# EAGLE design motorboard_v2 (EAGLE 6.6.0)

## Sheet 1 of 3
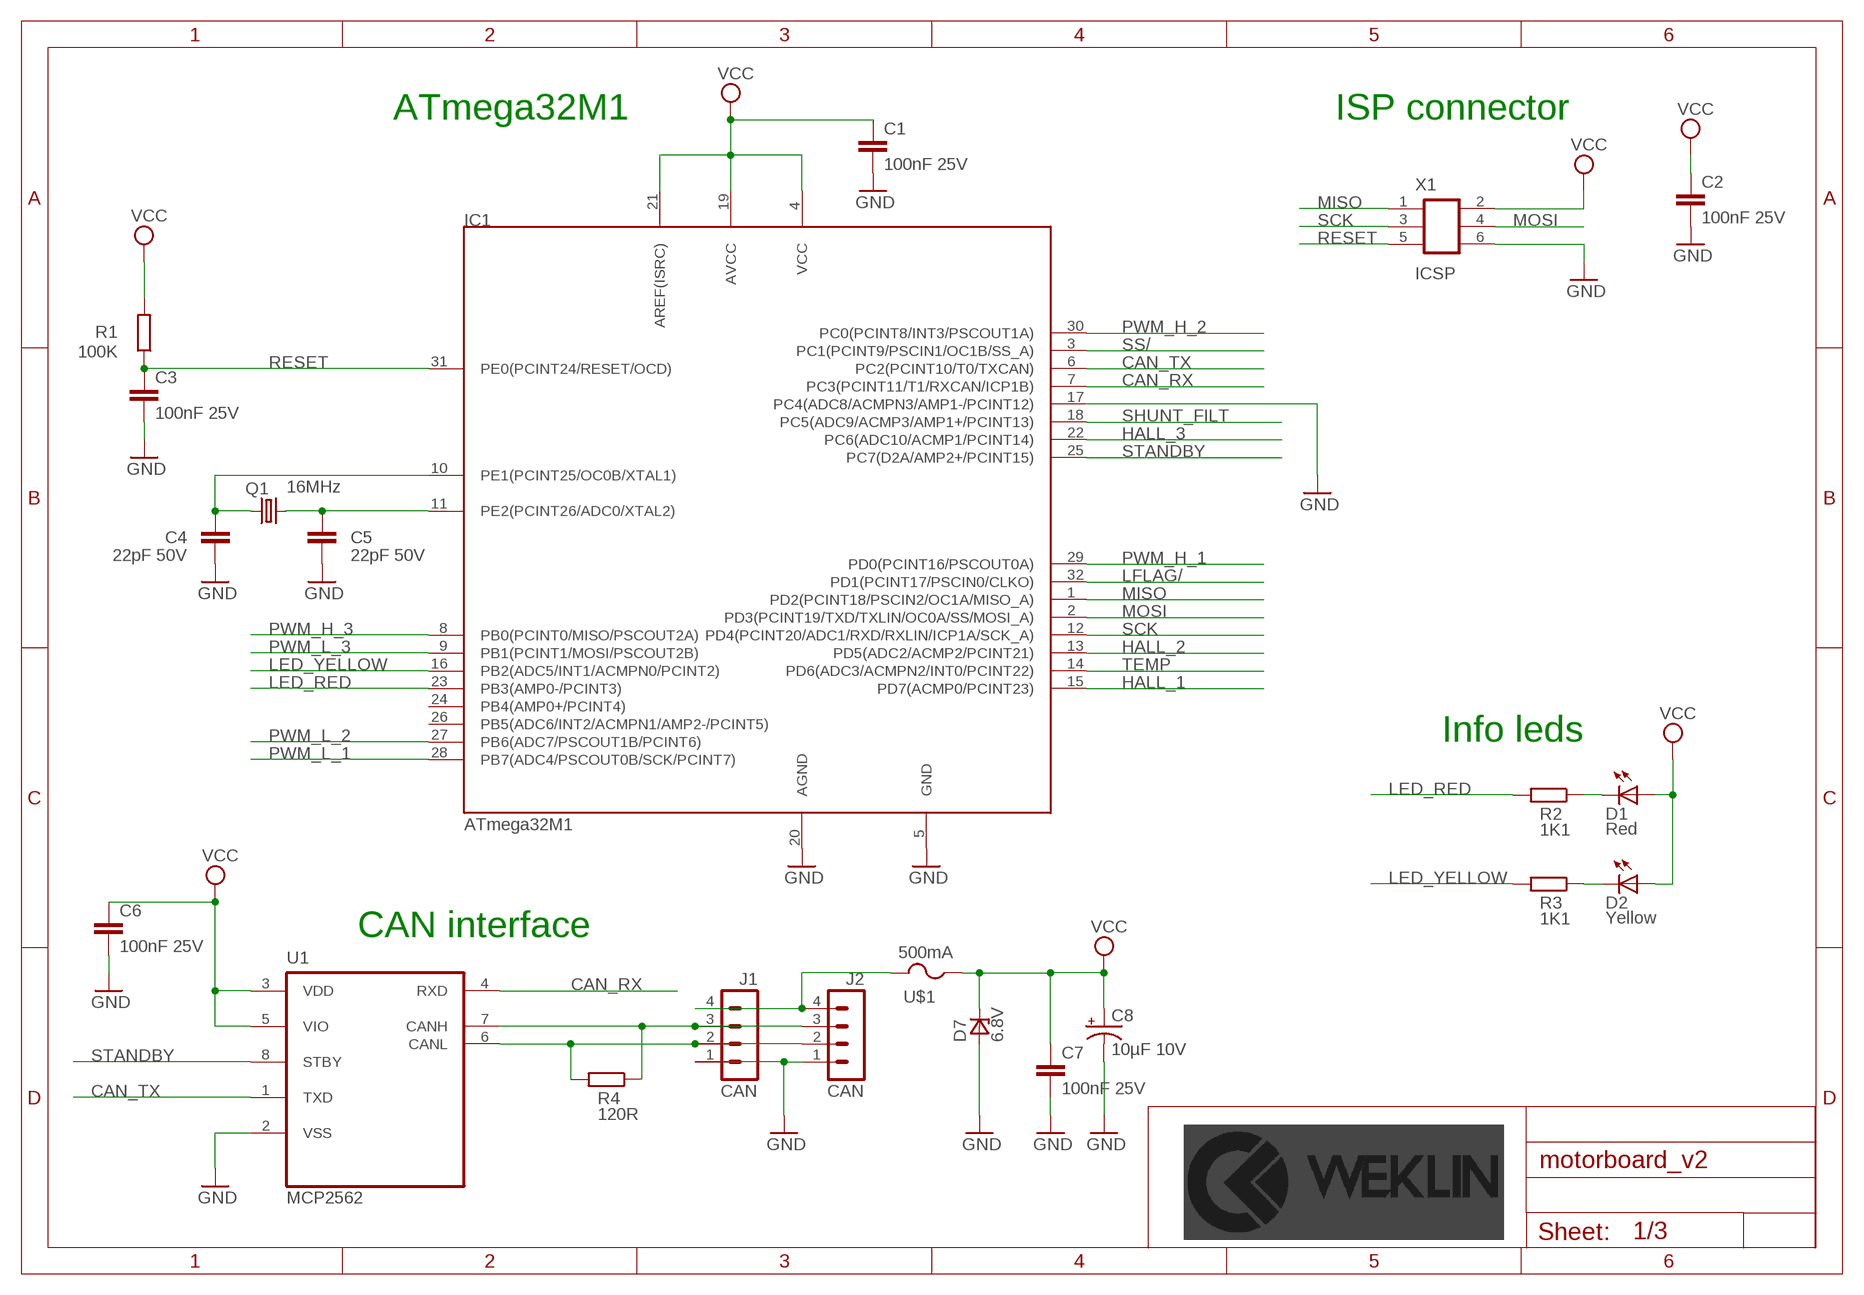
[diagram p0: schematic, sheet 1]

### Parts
C1  100nF 25V  CAPACITOR_NON_POL-100NF-25V(+-10%)(2012)  [C2012]
C2  100nF 25V  CAPACITOR_NON_POL-100NF-25V(+-10%)(2012)  [C2012]
C3  100nF 25V  CAPACITOR_NON_POL-100NF-25V(+-10%)(2012)  [C2012]
C4  22pF 50V  CAPACITOR_NON_POL-22PF-50V(+-5%)(2012)  [C2012]
C5  22pF 50V  CAPACITOR_NON_POL-22PF-50V(+-5%)(2012)  [C2012]
C6  100nF 25V  CAPACITOR_NON_POL-100NF-25V(+-10%)(2012)  [C2012]
C7  100nF 25V  CAPACITOR_NON_POL-100NF-25V(+-10%)(2012)  [C2012]
C8  10µF 10V  CAPACITOR_POL-10µF-10V(+-10%)(3216)  [EIA3216]
D1  Red  LEDVLDS1235G  [VLD]
D2  Yellow  LED-VLDY1235G  [VLD]
D7  6.8V  ZENER_UNIDIR6.8  [DO-214AA]
IC1  ATmega32M1  ATMEGA32M1-TQFP32  [TQFP32]
J1  CAN  MICROLOCK-4CMS_HORIZONTAL  [504195-0470]
J2  CAN  MICROLOCK-4CMS_HORIZONTAL  [504195-0470]
Q1  16MHz  CRYSTAL-16MHZ_SMD(3225)  [SMD_KX7]
R1  100K  RESISTOR-100K(+-1%)(2012)  [R2012]
R2  1K1  RESISTOR-1K1(+-1%)(2012)  [R2012]
R3  1K1  RESISTOR-1K1(+-1%)(2012)  [R2012]
R4  120R  RESISTOR-120R(+-1%)(2012)  [R2012]
U1  MCP2562  MCP2562-E/SN-SOIC8  [SOIC8]
U$1  500mA  FUSE0451.500MRL  [EIARS-481-2]
X1  ICSP  CON_2X3-SMD_1.27MM_FEMALE  [2X3_1.27_FEMALE_SMD]

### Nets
CAN_RX: IC1.7(PC3(PCINT11/T1/RXCAN/ICP1B)) U1.4(RXD)
CAN_TX: IC1.6(PC2(PCINT10/T0/TXCAN)) U1.1(TXD)
GND: C1.2 C2.2 C3.2 C4.2 C5.2 C6.2 C7.2 C8.C(-) D7.A IC1.5(GND) IC1.17(PC4(ADC8/ACMPN3/AMP1-/PCINT12)) IC1.20(AGND) J1.1 J2.1 U1.2(VSS) X1.6 ; also sheet 2,3
HALL_1: IC1.15(PD7(ACMP0/PCINT23)) ; also sheet 2
HALL_2: IC1.13(PD5(ADC2/ACMP2/PCINT21)) ; also sheet 2
HALL_3: IC1.22(PC6(ADC10/ACMP1/PCINT14)) ; also sheet 2
LED_RED: IC1.23(PB3(AMP0-/PCINT3)) R2.2
LED_YELLOW: IC1.16(PB2(ADC5/INT1/ACMPN0/PCINT2)) R3.2
LFLAG/: IC1.32(PD1(PCINT17/PSCIN0/CLKO)) ; also sheet 2
MISO: IC1.1(PD2(PCINT18/PSCIN2/OC1A/MISO_A)) X1.1 ; also sheet 2
MOSI: IC1.2(PD3(PCINT19/TXD/TXLIN/OC0A/SS/MOSI_A)) X1.4 ; also sheet 2
N$2: D1.C R2.1
N$3: D2.C R3.1
N$4: J1.4 J2.4 U$1.2
N$5: J1.2 J2.2 R4.2 U1.6(CANL)
N$6: J1.3 J2.3 R4.1 U1.7(CANH)
N$7: C5.1 IC1.11(PE2(PCINT26/ADC0/XTAL2)) Q1.3
N$9: C4.1 IC1.10(PE1(PCINT25/OC0B/XTAL1)) Q1.1
PWM_H_1: IC1.29(PD0(PCINT16/PSCOUT0A)) ; also sheet 3
PWM_H_2: IC1.30(PC0(PCINT8/INT3/PSCOUT1A)) ; also sheet 3
PWM_H_3: IC1.8(PB0(PCINT0/MISO/PSCOUT2A)) ; also sheet 3
PWM_L_1: IC1.28(PB7(ADC4/PSCOUT0B/SCK/PCINT7)) ; also sheet 3
PWM_L_2: IC1.27(PB6(ADC7/PSCOUT1B/PCINT6)) ; also sheet 3
PWM_L_3: IC1.9(PB1(PCINT1/MOSI/PSCOUT2B)) ; also sheet 3
RESET: C3.1 IC1.31(PE0(PCINT24/RESET/OCD)) R1.1 X1.5
SCK: IC1.12(PD4(PCINT20/ADC1/RXD/RXLIN/ICP1A/SCK_A)) X1.3 ; also sheet 2
SHUNT_FILT: IC1.18(PC5(ADC9/ACMP3/AMP1+/PCINT13)) ; also sheet 2
SS/: IC1.3(PC1(PCINT9/PSCIN1/OC1B/SS_A)) ; also sheet 2
STANDBY: IC1.25(PC7(D2A/AMP2+/PCINT15)) U1.8(STBY) ; also sheet 2
TEMP: IC1.14(PD6(ADC3/ACMPN2/INT0/PCINT22)) ; also sheet 2
VCC: C1.1 C2.1 C6.1 C7.1 C8.A(+) D1.A D2.A D7.C IC1.4(VCC) IC1.19(AVCC) IC1.21(AREF(ISRC)) R1.2 U1.3(VDD) U1.5(VIO) U$1.1 X1.2 ; also sheet 2
Unconnected: IC1.24(PB4(AMP0+/PCINT4)) IC1.26(PB5(ADC6/INT2/ACMPN1/AMP2-/PCINT5))

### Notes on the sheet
- ATmega32M1 | ISP connector
- Info leds
- CAN interface

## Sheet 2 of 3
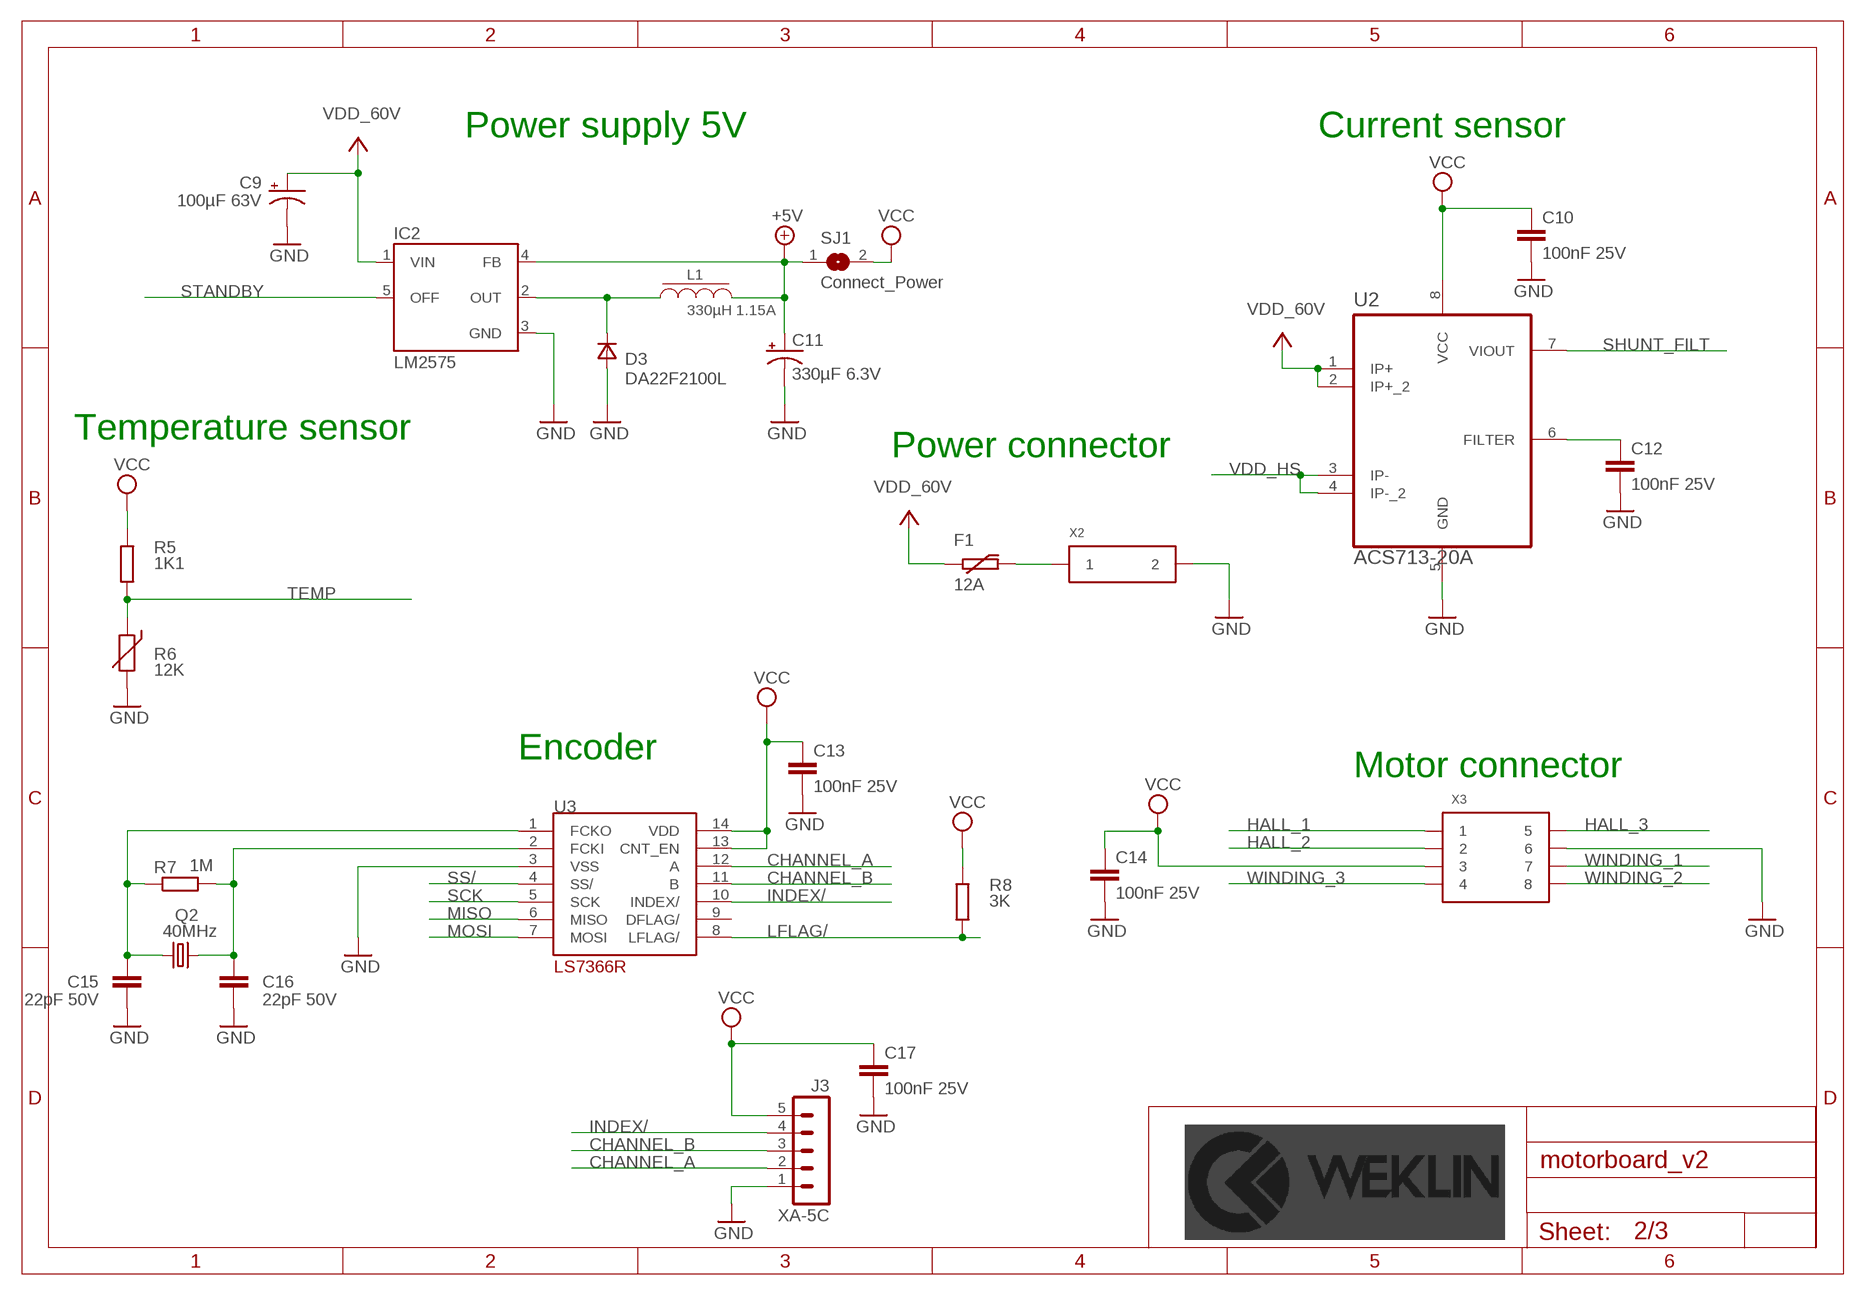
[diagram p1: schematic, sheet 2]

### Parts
C9  100µF 63V  CAPACITOR_POL-100µF-63V(+-10%)(1010)  [153CLV-1010]
C10  100nF 25V  CAPACITOR_NON_POL-100NF-25V(+-10%)(2012)  [C2012]
C11  330µF 6.3V  CAPACITOR_POL-330µF-6.3V(+-10%)(7343)  [EIA7343]
C12  100nF 25V  CAPACITOR_NON_POL-100NF-25V(+-10%)(2012)  [C2012]
C13  100nF 25V  CAPACITOR_NON_POL-100NF-25V(+-10%)(2012)  [C2012]
C14  100nF 25V  CAPACITOR_NON_POL-100NF-25V(+-10%)(2012)  [C2012]
C15  22pF 50V  CAPACITOR_NON_POL-22PF-50V(+-5%)(2012)  [C2012]
C16  22pF 50V  CAPACITOR_NON_POL-22PF-50V(+-5%)(2012)  [C2012]
C17  100nF 25V  CAPACITOR_NON_POL-100NF-25V(+-10%)(2012)  [C2012]
D3  DA22F2100L  DIODE-DA22F2100L  [SOD323]
F1  12A  PTCFUSE-12A-3216(1206)  [F3216]
IC2  LM2575  LM2575-TO263  [TO263-5]
J3  XA-5C  XA-5-RIGHT_ANGLE  [S05B-XASK-1]
L1  330µH 1.15A  SRR1260A-331K  [DRA124]
Q2  40MHz  CRYSTAL-40MHZ_SMD(3225)  [SMD_KX7]
R5  1K1  RESISTOR-1K1(+-1%)(2012)  [R2012]
R6  12K  NB12L00123KBB-2012(0805)  [T2012]
R7  1M  RESISTOR-1M(+-1%)(2012)  [R2012]
R8  3K  RESISTOR-3K(+-1%)(2012)  [R2012]
SJ1  Connect_Power  JUMPER_PCB  [SJ]
U2  ACS713-20A  ASC713713ELCTR-20A-T  [SOIC8]
U3  LS7366R  LS7366R-TS-TSSOP14  [TSSOP14]
X2  Mini-Fit  MINI-FIT-JR-025569-NA1  [5569-02]
X3  Mini-Fit  MINI-FIT-JR-085569-NA1  [5569-08]

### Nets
+5V: C11.A(+) IC2.4(FB) L1.2 SJ1.1 ; also sheet 3
CHANNEL_A: J3.2 U3.12(A)
CHANNEL_B: J3.3 U3.11(B)
GND: C9.- C10.2 C11.C(-) C12.2 C13.2 C14.2 C15.2 C16.2 C17.2 D3.2(A) IC2.3(GND) J3.1 R6.2 U2.5(GND) U3.3(VSS) X2.P2 X3.P6 ; also sheet 1,3
HALL_1: X3.P1 ; also sheet 1
HALL_2: X3.P2 ; also sheet 1
HALL_3: X3.P5 ; also sheet 1
INDEX/: J3.4 U3.10(INDEX/)
LFLAG/: R8.2 U3.8(LFLAG/) ; also sheet 1
MISO: U3.6(MISO) ; also sheet 1
MOSI: U3.7(MOSI) ; also sheet 1
N$1: D3.1(C) IC2.2(OUT) L1.1
N$11: C16.1 Q2.3 R7.2 U3.2(FCKI)
N$14: C15.1 Q2.1 R7.1 U3.1(FCKO)
N$15: F1.2 X2.P1
N$16: C12.1 U2.6(FILTER)
SCK: U3.5(SCK) ; also sheet 1
SHUNT_FILT: U2.7(VIOUT) ; also sheet 1
SS/: U3.4(SS/) ; also sheet 1
STANDBY: IC2.5(OFF) ; also sheet 1
TEMP: R5.1 R6.1 ; also sheet 1
VCC: C10.1 C13.1 C14.1 C17.1 J3.5 R5.2 R8.1 SJ1.2 U2.8(VCC) U3.13(CNT_EN) U3.14(VDD) X3.P3 ; also sheet 1
VDD: C9.+ F1.1 IC2.1(VIN) U2.1(IP+) U2.2(IP+_2) ; supply symbol labelled VDD_60V
VDD_HS: U2.3(IP-) U2.4(IP-_2) ; also sheet 3
WINDING_1: X3.P7 ; also sheet 3
WINDING_2: X3.P8 ; also sheet 3
WINDING_3: X3.P4 ; also sheet 3
Unconnected: U3.9(DFLAG/)

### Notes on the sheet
- Power supply 5V | Current sensor
- Temperature sensor
- Power connector
- Encoder
- Motor connector

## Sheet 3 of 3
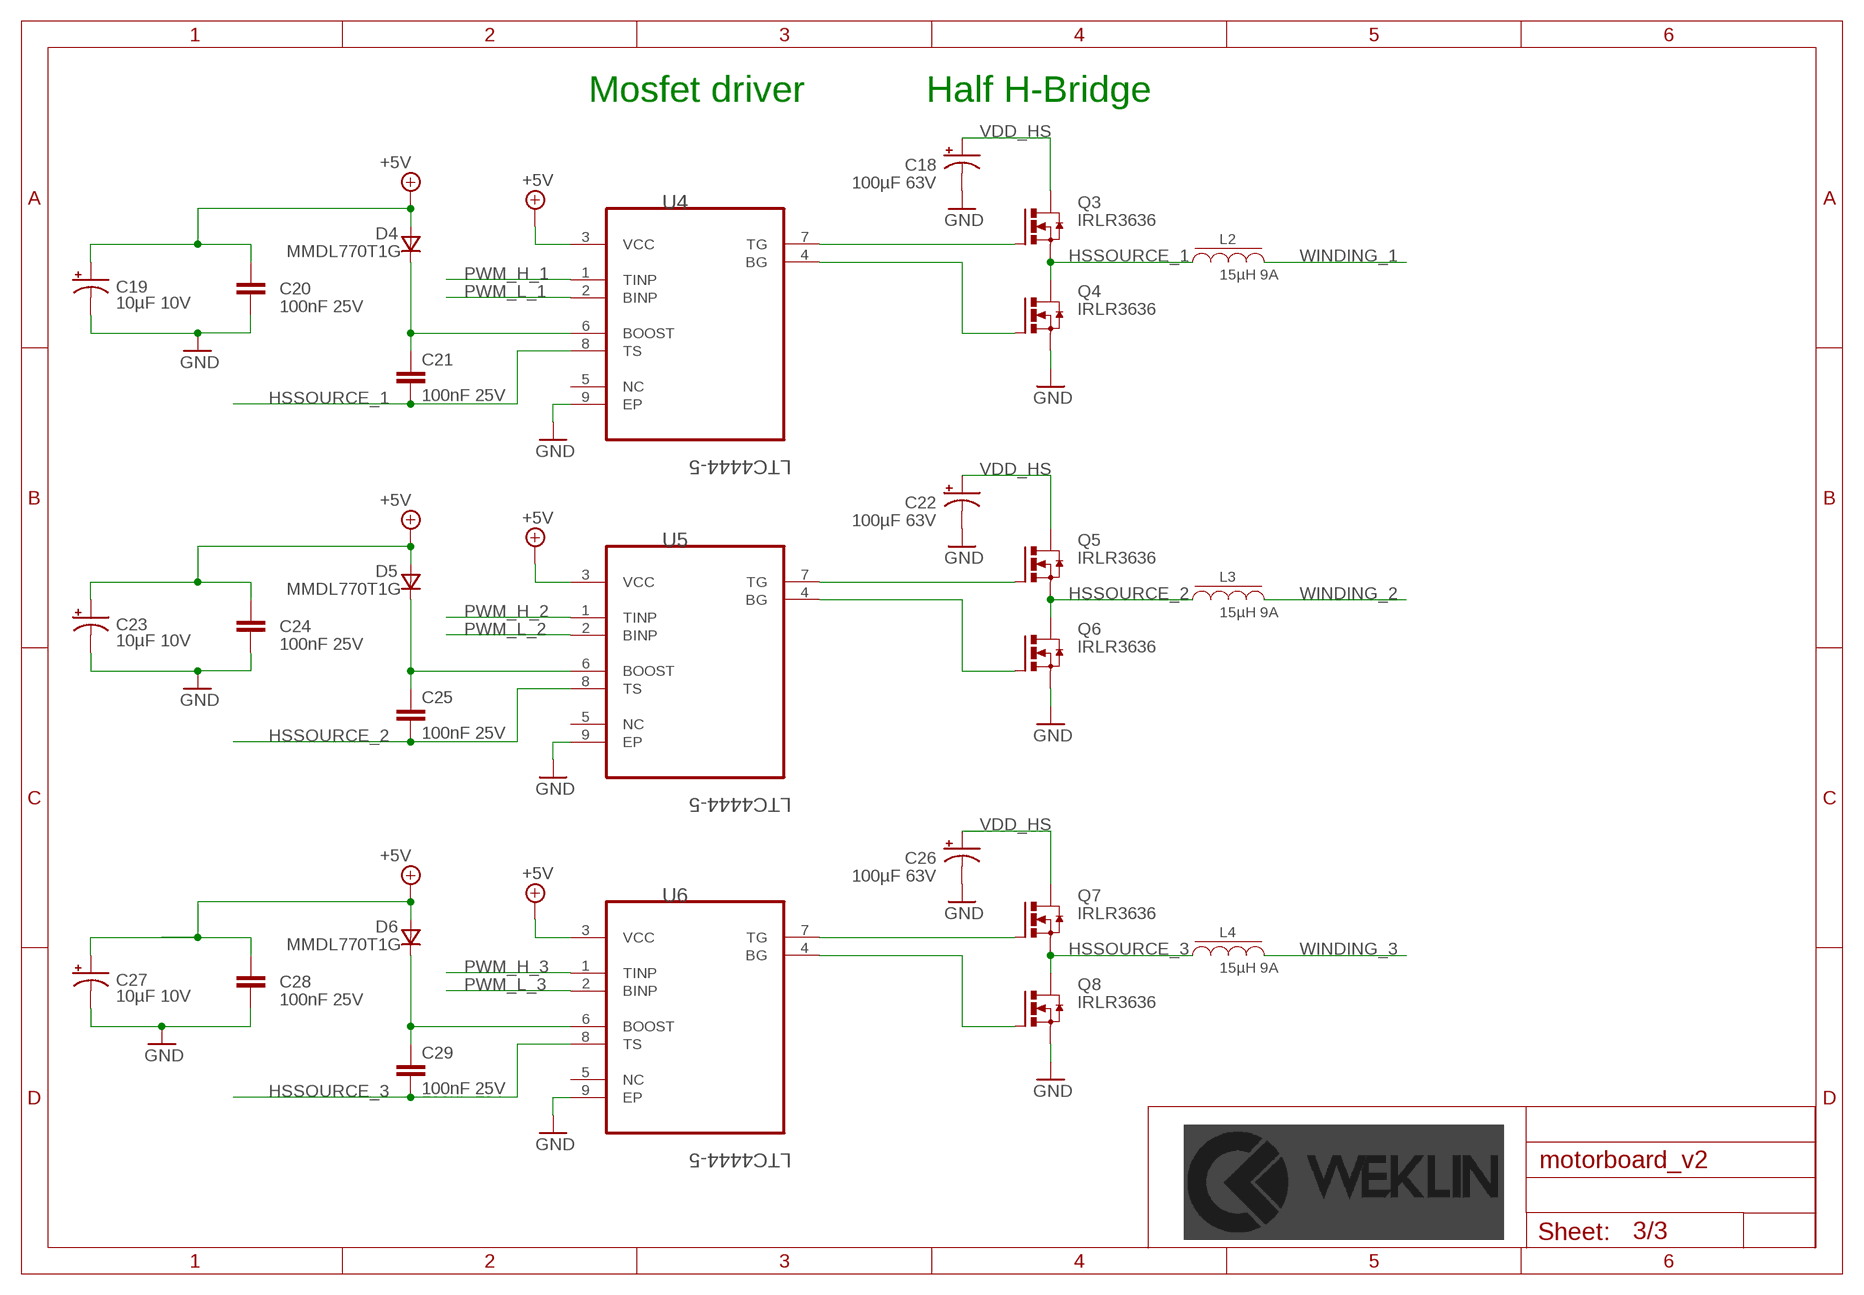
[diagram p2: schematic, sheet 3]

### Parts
C18  100µF 63V  CAPACITOR_POL-100µF-63V(+-10%)(1010)  [153CLV-1010]
C19  10µF 10V  CAPACITOR_POL-10µF-10V(+-10%)(3216)  [EIA3216]
C20  100nF 25V  CAPACITOR_NON_POL-100NF-25V(+-10%)(2012)  [C2012]
C21  100nF 25V  CAPACITOR_NON_POL-100NF-25V(+-10%)(2012)  [C2012]
C22  100µF 63V  CAPACITOR_POL-100µF-63V(+-10%)(1010)  [153CLV-1010]
C23  10µF 10V  CAPACITOR_POL-10µF-10V(+-10%)(3216)  [EIA3216]
C24  100nF 25V  CAPACITOR_NON_POL-100NF-25V(+-10%)(2012)  [C2012]
C25  100nF 25V  CAPACITOR_NON_POL-100NF-25V(+-10%)(2012)  [C2012]
C26  100µF 63V  CAPACITOR_POL-100µF-63V(+-10%)(1010)  [153CLV-1010]
C27  10µF 10V  CAPACITOR_POL-10µF-10V(+-10%)(3216)  [EIA3216]
C28  100nF 25V  CAPACITOR_NON_POL-100NF-25V(+-10%)(2012)  [C2012]
C29  100nF 25V  CAPACITOR_NON_POL-100NF-25V(+-10%)(2012)  [C2012]
D4  MMDL770T1G  DIODE-MMDL770T1G  [SOD323]
D5  MMDL770T1G  DIODE-MMDL770T1G  [SOD323]
D6  MMDL770T1G  DIODE-MMDL770T1G  [SOD323]
L2  15µH 9A  SRP1265A-150M  [DRA127]
L3  15µH 9A  SRP1265A-150M  [DRA127]
L4  15µH 9A  SRP1265A-150M  [DRA127]
Q3  IRLR3636  [TO252]
Q4  IRLR3636  [TO252]
Q5  IRLR3636  [TO252]
Q6  IRLR3636  [TO252]
Q7  IRLR3636  [TO252]
Q8  IRLR3636  [TO252]
U4  LTC4444-5  [MSOP8]
U5  LTC4444-5  [MSOP8]
U6  LTC4444-5  [MSOP8]

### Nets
+5V: C19.A(+) C20.1 C23.A(+) C24.1 C27.A(+) C28.1 D4.2(A) D5.2(A) D6.2(A) U4.3(VCC) U5.3(VCC) U6.3(VCC) ; also sheet 2
GND: C18.- C19.C(-) C20.2 C22.- C23.C(-) C24.2 C26.- C27.C(-) C28.2 Q4.3(S) Q6.3(S) Q8.3(S) U4.9(EP) U5.9(EP) U6.9(EP) ; also sheet 1,2
HSSOURCE_1: C21.2 L2.1 Q3.3(S) Q4.4(D) U4.8(TS)
HSSOURCE_2: C25.2 L3.1 Q5.3(S) Q6.4(D) U5.8(TS)
HSSOURCE_3: C29.2 L4.1 Q7.3(S) Q8.4(D) U6.8(TS)
N$8: C25.1 D5.1(C) U5.6(BOOST)
N$10: C21.1 D4.1(C) U4.6(BOOST)
N$12: Q4.1(G) U4.4(BG)
N$13: Q3.1(G) U4.7(TG)
N$17: Q6.1(G) U5.4(BG)
N$18: Q5.1(G) U5.7(TG)
N$20: C29.1 D6.1(C) U6.6(BOOST)
N$21: Q8.1(G) U6.4(BG)
N$22: Q7.1(G) U6.7(TG)
PWM_H_1: U4.1(TINP) ; also sheet 1
PWM_H_2: U5.1(TINP) ; also sheet 1
PWM_H_3: U6.1(TINP) ; also sheet 1
PWM_L_1: U4.2(BINP) ; also sheet 1
PWM_L_2: U5.2(BINP) ; also sheet 1
PWM_L_3: U6.2(BINP) ; also sheet 1
VDD_HS: C18.+ C22.+ C26.+ Q3.4(D) Q5.4(D) Q7.4(D) ; also sheet 2
WINDING_1: L2.2 ; also sheet 2
WINDING_2: L3.2 ; also sheet 2
WINDING_3: L4.2 ; also sheet 2
Unconnected: U4.5(NC) U5.5(NC) U6.5(NC)

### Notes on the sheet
- Mosfet driver | Half H-Bridge

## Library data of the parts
C1-C3 C6 C7 C10 C12-C14 C17 C20 C21 C24 C25 C28 C29 = weklin_capacitor:CAPACITOR_NON_POL: Condensateur céramique multicouche; LIB: weklin_capacitor; MANUFACTURER: AVX; MPN: 08053C104KAT2A; OC_FARNELL: 2280951; PRICE: 0,0036
C4 C5 C15 C16 = weklin_capacitor:CAPACITOR_NON_POL: Condensateur céramique multicouche; LIB: weklin_capacitor; MANUFACTURER: Multicomp; MPN: MC0805N220J500CT; OC_FARNELL: 2310684; PRICE: 0,0078
C8 C19 C23 C27 = weklin_capacitor:CAPACITOR_POL: Capacitor; LIB: weklin_capacitor; MANUFACTURER: Kemet; MPN: T491A106K010AT; OC_FARNELL: 2250086; PRICE: 0,0578
C9 C18 C22 C26 = weklin_capacitor:CAPACITOR_POL: Capacitor; LIB: weklin_capacitor; MANUFACTURER: Nichicon; MPN: UUX1J101MNL1GS; OC_FARNELL: 1898746; PRICE: 0,45
C11 = weklin_capacitor:CAPACITOR_POL: Capacitor; LIB: weklin_capacitor; MANUFACTURER: Kemet; MPN: T491D337K006AT; OC_FARNELL: 2313928; PRICE: 0,497
D1 = weklin_led:LED: Led; LIB: weklin_led; MANUFACTURER: Vishay; MPN: VLDS1235G; OC_FARNELL: 2494682; PRICE: 0,003
D2 = weklin_led:LED: Led; LIB: weklin_led; MANUFACTURER: Vishay; MPN: VLDY1235G; OC_FARNELL: 2494684; PRICE: 0,003
D3 = weklin_diode:DIODE: Diode; LIB: weklin_diode; MPN: DA22F2100L; OC_FARNELL: 2459014; PRICE: 0,29
D4-D6 = weklin_diode:DIODE: Diode; LIB: weklin_diode; MPN: MMDL770T1G; OC_FARNELL: 2317690; PRICE: 0,034
D7 = weklin_diode:ZENER_UNIDIR: P6SMBxxA Series of unidirectional Transient Voltage Suppressor Diodes; LIB: weklin_diode; MANUFACTURER: ON Semiconductor; MPN: P6SMB6.8AT3G; OC_FARNELL: 1459166RL; PRICE: 0,178
F1 = weklin_fuse:PTCFUSE: Fuse time lag; LIB: weklin_fuse; MANUFACTURER: Schruter; MPN: 3413.0329.22; OC_FARNELL: 1829472; PRICE: 0,973
IC1 = weklin_micro-atmell:ATMEGA32M1: ATMEL ATMEGA32M1-AU MCU 8 BITS ATMEGA 16MHZ; LIB: weklin_micro_atmell; MANUFACTURER: Atmel; MPN: ATmega32M1-AU; OC_FARNELL: 2443180; PRICE: 6,18
IC2 = weklin_regulator:LM2575: SIMPLE SWITCHER 1A Step-Down Voltage Regulator; LIB: weklin_regulator; MPN: LM2575HVS-5.0/NOPB; OC_FARNELL: 1469170; PRICE: 5,04
J1 J2 = weklin_micro-lock:MICROLOCK-4: Connecteur MOLEX de 4 Contacts Série Mini50 GEII/IUT ANGERS; LIB: weklin_micro-lock; MANUFACTURER: Molex; MPN: 504195-0470; OC_FARNELL: 2445490; PRICE: 0,713
J3 = weklin_xa:XA-5: Connector JST XA 5 way; LIB: weklin_xa; MPN: S05B-XASK-1(LF)(SN); OC_FARNELL: 9492160; PRICE: 0,546
L1 = weklin_inductor:SRR1260A-331K: Power inductor 330µH 1.15A; LIB: weklin_inductor; MPN: SRR1260A-331K; OC_FARNELL: 2374141; PRICE: 1,04
L2-L4 = weklin_inductor:SRP1265A-150M: Power inductor 15µH 9A; LIB: weklin_inductor; MPN: SRP1265A-150M; OC_FARNELL: 2434073; PRICE: 1,20
Q1 = weklin_crystal:CRYSTAL: Crystal resonator; LIB: weklin_crystal; MANUFACTURER: AEL CRYSTALS; MPN: E3SB16.0000F09G11AE; OC_FARNELL: 2467444RL; PRICE: 0,315
Q2 = weklin_crystal:CRYSTAL: Crystal resonator; LIB: weklin_crystal; MANUFACTURER: Epson; MPN: X1E0000210488 TSX-3225; OC_FARNELL: 2471834; PRICE: 0,636
Q3-Q8 = weklin_mosfet:IRLR3636: Transistor MOSFET, Canal N; LIB: weklin_mosfet; MANUFACTURER: International Rectifier; MPN: IRLR3636PbF; OC_FARNELL: 1698302; PRICE: 1,89
R1 = weklin_resistor:RESISTOR: Resistor; LIB: weklin_resistor; MANUFACTURER: Multicomp; MPN: MCWR08X1003FTL; OC_FARNELL: 2446868; PRICE: 0,0014
R2 R3 R5 = weklin_resistor:RESISTOR: Resistor; LIB: weklin_resistor; MANUFACTURER: Multicomp; MPN: MC0805S8F1101T5E; OC_FARNELL: 1635316; PRICE: 0,003
R4 = weklin_resistor:RESISTOR: Resistor; LIB: weklin_resistor; MANUFACTURER: Multicomp; MPN: MCWR08X1200FTL; OC_FARNELL: 2446878; PRICE: 0,0014
R6 = weklin_thermistor:NB12L00123KBB: Thermistor; LIB: weklin_thermistor; MPN: NB12L00123KBB; OC_FARNELL: 1672292; PRICE: 0,14
R7 = weklin_resistor:RESISTOR: Resistor; LIB: weklin_resistor; MPN: MCWR08X1004FTL; OC_FARNELL: 2446913; PRICE: 0,0014
R8 = weklin_resistor:RESISTOR: Resistor; LIB: weklin_resistor; MPN: MC0805S8F3001T5E; OC_FARNELL: 1635321; PRICE: 0,003
SJ1 = weklin_jumper:JUMPER_PCB: SMD solder JUMPER; LIB: weklin_jumper; MPN: N.A.; OC_FARNELL: N.A.; PRICE: 0
U1 = weklin_ic_can:MCP2562-E/SN: High-Speed CAN Transceiver; LIB: weklin_ic_can; MANUFACTURER: Microchip; MPN: MCP2562-E/SN; OC_FARNELL: 2362839; PRICE: 1,12
U2 = weklin_sensor:ASC713: Linear Current Sensor; LIB: weklin_sensor; MPN: ACS713ELCTR-20A-T; OC_FARNELL: 1651976; PRICE: 4,44
U3 = weklin_ic_special:LS7366R-TS: 32-bits quadrature counter IC with SPI; LIB: weklin_ic_special; MPN: LS7366R-TS; OC_FARNELL: N.A.; PRICE: 5
U4-U6 = weklin_mosfet_driver:LTC4444: High Voltage Synchronous N-Channel MOSFET Driver; LIB: weklin_mosfet_driver; MPN: LTC4444EMS8E-5#PBF; OC_FARNELL: 2294863; PRICE: 3,5
U$1 = weklin_fuse:FUSE: Fuse; LIB: weklin_fuse; MANUFACTURER: Littlefuse; MPN: 0451500MRL; OC_FARNELL: 2383271; PRICE: 0,527
X1 = weklin_connector:CON_2X3: Board-To-Board Connector, Micro-MaTch Series, Embase, 6voies.; LIB: weklin_connector; MANUFACTURER: AMPHENOL FCI; MPN: 20021321-00006C4LF; OC_FARNELL: 1865307; PRICE: 0,52
X2 = weklin_mini-fit:MINI-FIT-JR-02: Mini-Fit Jr connector 2 way; LIB: weklin_mini-fit; MANUFACTURER: Molex; MPN: 39-29-1028; OC_FARNELL: 1012166; PRICE: 0,506
X3 = weklin_mini-fit:MINI-FIT-JR-08: Mini-Fit Jr connector 8 way; LIB: weklin_mini-fit; MANUFACTURER: MOLEX; MPN: 39-29-1088; OC_FARNELL: 9732160; PRICE: 1,27

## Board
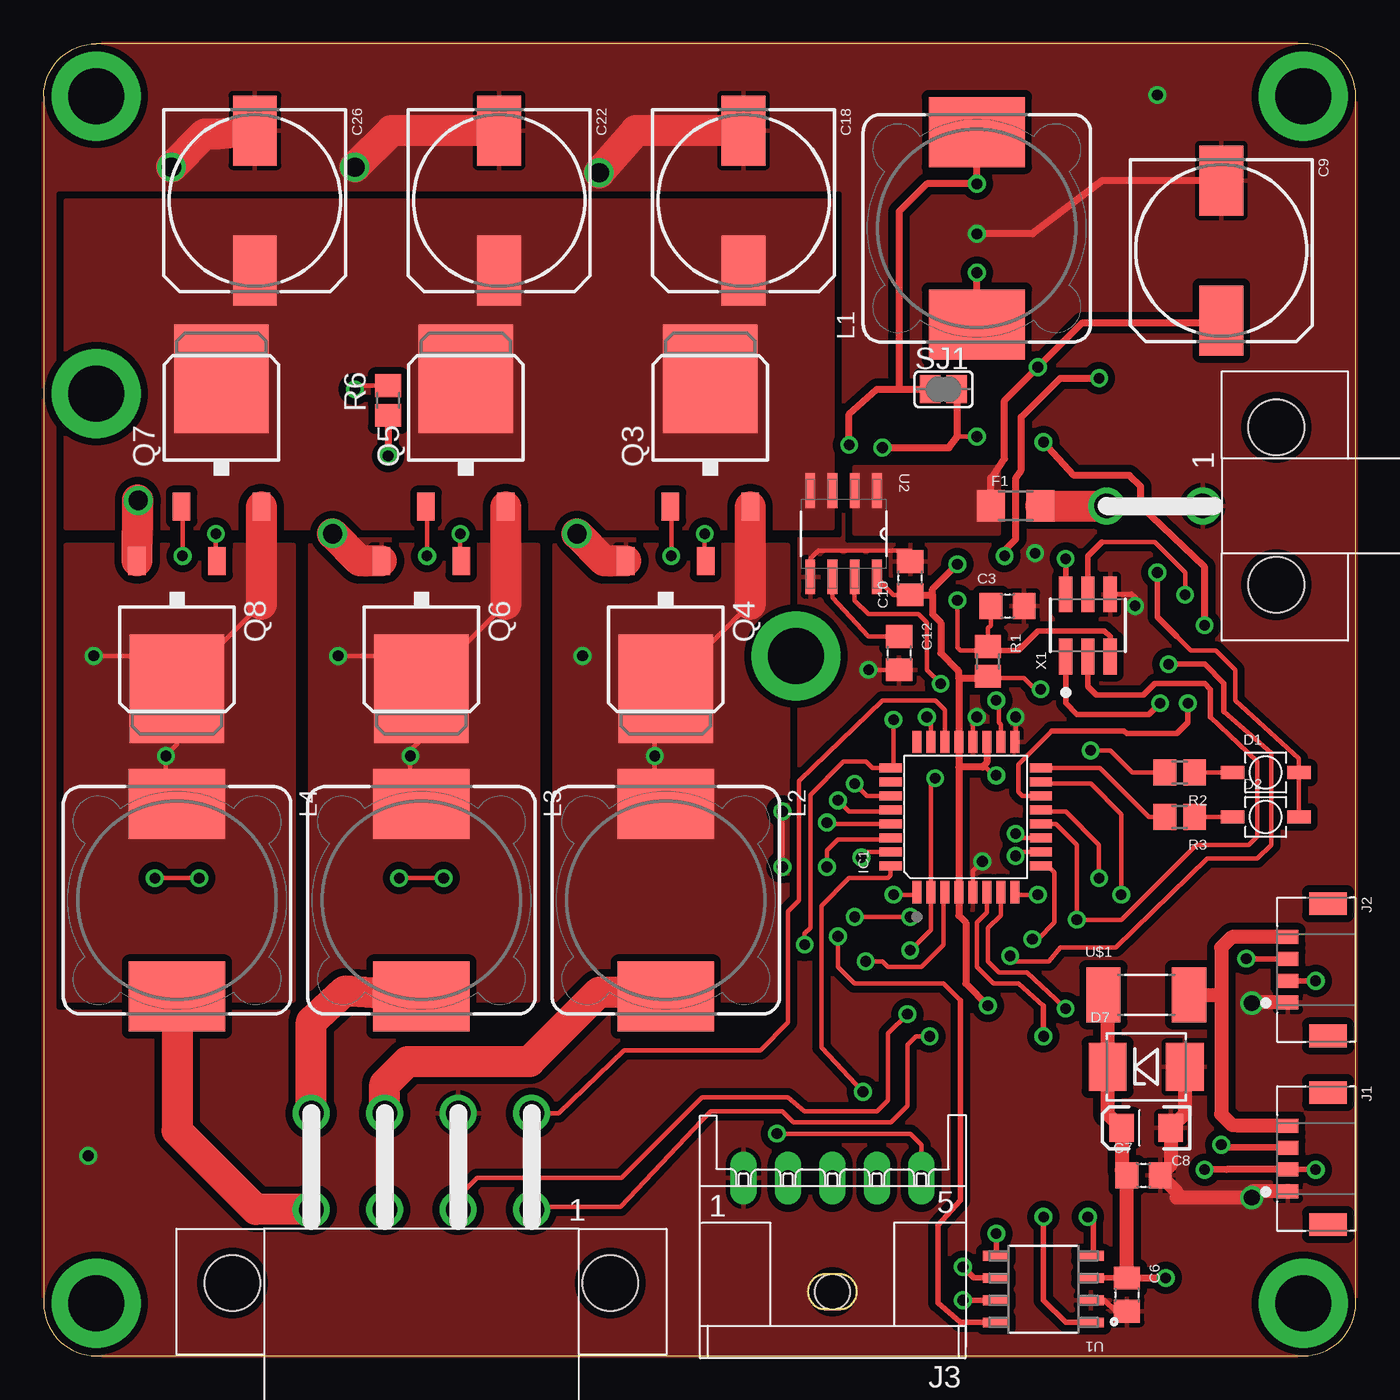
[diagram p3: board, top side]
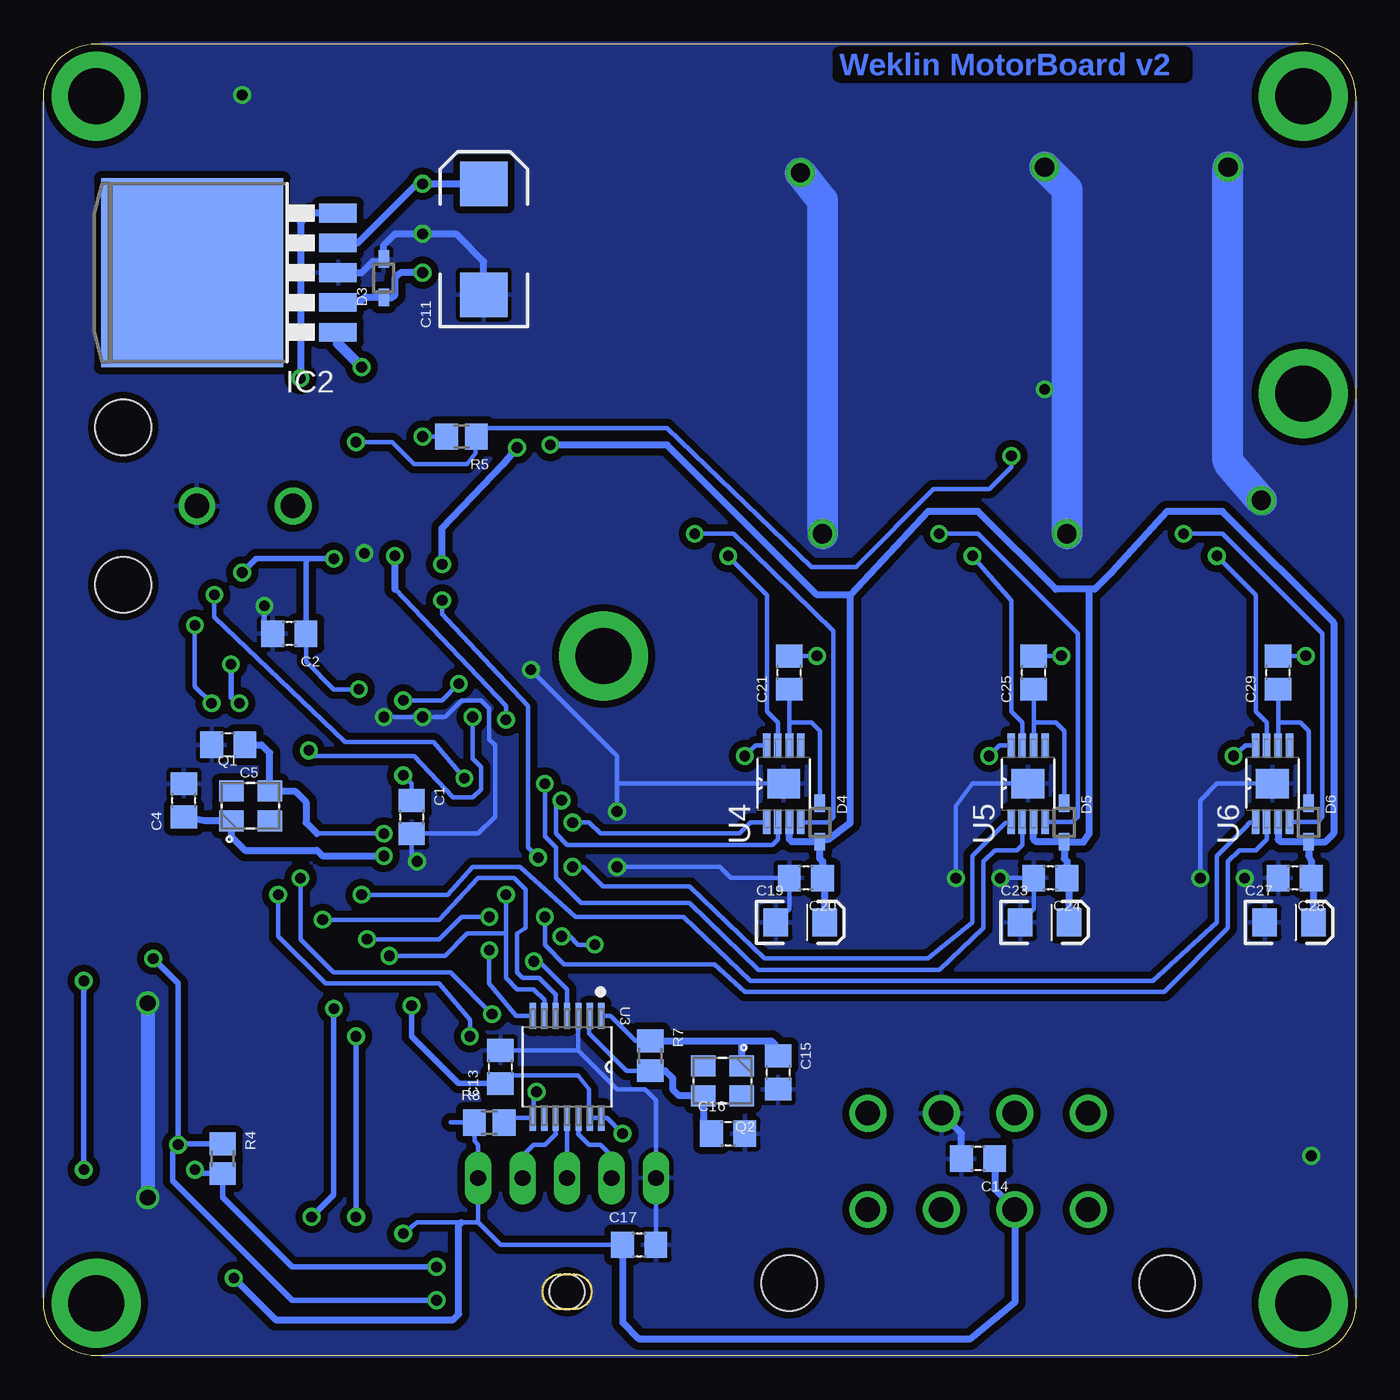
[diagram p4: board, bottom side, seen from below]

Size 75 x 75 mm. Coordinates in mm from the lower left corner, seen from the top.
Outline: 3,0 72,0 arc90 75,3 75,72 arc90 72,75 3,75 arc90 0,72 0,3 arc90 3,0
Copper layers ((1*2)+(15*16)): Top 0.035mm / dielectric 0.489mm / Route2 0.035mm / dielectric 0.486mm / Route15 0.035mm / dielectric 0.486mm / Bottom 0.035mm
Design rules "default *": minimum track width 10mil, minimum drill 24mil, track to track 8mil, track to pad 8mil, pad to pad 8mil, via to via 8mil, smd to smd 8mil, copper to edge 0mil, drill to drill 8mil, minimum pad ring 10mil, minimum via ring 8mil, stop-mask expansion 4mil, vias tented up to drill 0mil, thermal gap 10mil

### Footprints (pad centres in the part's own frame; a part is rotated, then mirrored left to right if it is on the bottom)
C2012 = smd 1.3 x 1.5: 1 -0.95,0; 2 0.95,0
EIA3216 = smd 1.4 x 1.6: A 1.4,0; C -1.4,0
153CLV-1010 = smd 4 x 2.5: + 4,0; - -4,0
EIA7343 = smd 2.55 x 2.7: A 3.17,0; C -3.17,0
VLD = smd 1.35 x 0.75: A 1.9,0; C -1.9,0
SOD323 = smd 1 x 0.6: 1 -1.1,0; 2 1.1,0
DO-214AA = smd 2.159 x 2.743: A 2.21,0; C -2.21,0
F3216 = smd 1.6 x 1.803: 1 -1.422,0; 2 1.422,0
TQFP32 = smd 1.27 x 0.508: 1 -4.293,2.8; 2 -4.293,2; 3 -4.293,1.2; 4 -4.293,0.4; 5 -4.293,-0.4; 6 -4.293,-1.2; 7 -4.293,-2; 8 -4.293,-2.8; 17 4.293,-2.8; 18 4.293,-2; 19 4.293,-1.2; 20 4.293,-0.4; 21 4.293,0.4; 22 4.293,1.2; 23 4.293,2; 24 4.293,2.8 | smd 0.508 x 1.27: 9 -2.8,-4.293; 10 -2,-4.293; 11 -1.2,-4.293; 12 -0.4,-4.293; 13 0.4,-4.293; 14 1.2,-4.293; 15 2,-4.293; 16 2.8,-4.293; 25 2.8,4.293; 26 2,4.293; 27 1.2,4.293; 28 0.4,4.293; 29 -0.4,4.293; 30 -1.2,4.293; 31 -2,4.293; 32 -2.8,4.293
TO263-5 = smd 1.067 x 2.159: 1 -3.404,-5.791; 2 -1.702,-5.791; 3 0,-5.791; 4 1.702,-5.791; 5 3.404,-5.791 | smd 10.8 x 10.41: 6 0,2.54
504195-0470 = smd 0.8 x 1.2: 1 1.875,0; 2 0.625,0; 3 -0.625,0; 4 -1.875,0 | smd 1.3 x 2.15: P$5 -3.775,2.295; P$6 3.775,2.295
S05B-XASK-1 = drill 0.9 pad 1.524 long: 1 5.08,-3.81; 2 2.54,-3.81; 3 0,-3.81; 4 -2.54,-3.81; 5 -5.08,-3.81 | hole 2: 0,2.69
DRA124 = smd 4 x 5.5: 1 -5.5,0; 2 5.5,0
DRA127 = smd 4 x 5.5: 1 -5.5,0; 2 5.5,0
SMD_KX7 = smd 1.4 x 1.2: 1 -1.1,-0.85; 2 1.1,-0.85; 3 1.1,0.85; 4 -1.1,0.85
TO252 = smd 1 x 1.6: 1 -2.28,-4.8; 3 2.28,-4.8 | smd 5.4 x 6.2: 4 0,2.5
R2012 = smd 1.3 x 1.5: 1 -0.85,0; 2 0.85,0
T2012 = smd 1.3 x 1.5: 1 -0.85,0; 2 0.85,0
SJ = smd 1.168 x 1.6: 1 -0.762,0; 2 0.762,0
SOIC8 = smd 1.473 x 0.559: 1 -2.718,1.905; 2 -2.718,0.635; 3 -2.718,-0.635; 4 -2.718,-1.905; 5 2.718,-1.905; 6 2.718,-0.635; 7 2.718,0.635; 8 2.718,1.905
SOIC8' = smd 1.981 x 0.559: 1 -2.464,1.905; 2 -2.464,0.635; 3 -2.464,-0.635; 4 -2.464,-1.905; 5 2.464,-1.905; 6 2.464,-0.635; 7 2.464,0.635; 8 2.464,1.905
TSSOP14 = smd 1.473 x 0.356: 1 -2.921,1.956; 2 -2.921,1.295; 3 -2.921,0.66; 4 -2.921,0; 5 -2.921,-0.66; 6 -2.921,-1.295; 7 -2.921,-1.956; 8 2.921,-1.956; 9 2.921,-1.295; 10 2.921,-0.66; 11 2.921,0; 12 2.921,0.66; 13 2.921,1.295; 14 2.921,1.956
MSOP8 = smd 1.397 x 0.432: 1 -2.184,0.965; 2 -2.184,0.33; 3 -2.184,-0.33; 4 -2.184,-0.965; 5 2.184,-0.965; 6 2.184,-0.33; 7 2.184,0.33; 8 2.184,0.965 | smd 1.676 x 1.88: 9 0,0
EIARS-481-2 = smd 1.956 x 3.15: 1 -2.451,0; 2 2.451,0
2X3_1.27_FEMALE_SMD = smd 2.05 x 0.76: 1 -1.775,1.27; 2 1.775,1.27; 3 -1.775,0; 4 1.775,0; 5 -1.775,-1.27; 6 1.775,-1.27
5569-02 = drill 1.4: P1 0,2.75; P2 0,-2.75 | hole 3.2: -4.5,-6.95; 4.5,-6.95
5569-08 = drill 1.4: P1 6.3,-2.75; P2 2.1,-2.75; P3 -2.1,-2.75; P4 -6.3,-2.75; P5 6.3,2.75; P6 2.1,2.75; P7 -2.1,2.75; P8 -6.3,2.75 | hole 3.2: -10.8,-6.95; 10.8,-6.95

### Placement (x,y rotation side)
C1  53.98,30.8 270 bottom
C2  60.96,41.27 180 bottom
C3  55.09,42.86 0 top
C4  66.99,31.75 90 bottom
C5  64.45,34.92 180 bottom
C6  61.91,3.49 270 top
C7  62.87,10.32 0 top
C8  63.02,13.02 180 top
C9  67.31,63.18 270 top
C10  49.53,44.45 90 top
C11  49.85,63.82 90 bottom
C12  48.9,40.16 270 top
C13  48.9,16.51 90 bottom
C14  21.59,11.27 180 bottom
C15  33.02,16.19 270 bottom
C16  35.88,12.7 0 bottom
C17  40.96,6.35 0 bottom
C18  40.01,66.04 270 top
C19  31.75,24.77 0 bottom
C20  31.43,27.3 180 bottom
C21  32.38,39.05 90 bottom
C22  26.04,66.04 270 top
C23  17.78,24.77 0 bottom
C24  17.46,27.3 180 bottom
C25  18.41,39.05 90 bottom
C26  12.06,66.04 270 top
C27  3.81,24.77 0 bottom
C28  3.49,27.3 180 bottom
C29  4.45,39.05 90 bottom
D1  69.85,33.34 0 top
D2  69.85,30.8 0 top
D3  55.56,61.59 90 bottom
D4  30.64,30.48 270 bottom
D5  16.67,30.48 270 bottom
D6  2.7,30.48 270 bottom
D7  63.02,16.51 0 top
F1  55.56,48.58 0 top
IC1  52.7,30.8 90 top
IC2  63.98,61.91 90 bottom
J1  71.12,11.27 270 top
J2  71.12,22.07 270 top
J3  45.09,6.35 180 top
L1  53.34,64.45 90 top
L2  35.56,26.04 270 top
L3  21.59,26.04 270 top
L4  7.62,26.04 270 top
Q1  63.18,31.43 0 bottom
Q2  36.2,15.72 180 bottom
Q3  38.1,53.34 0 top
Q4  35.56,40.64 180 top
Q5  24.13,53.34 0 top
Q6  21.59,40.64 180 top
Q7  10.16,53.34 0 top
Q8  7.62,40.64 180 top
R1  53.98,39.69 270 top
R2  64.93,33.34 180 top
R3  64.93,30.8 180 top
R4  64.77,11.27 270 bottom
R5  51.12,52.55 180 bottom
R6  19.68,54.61 90 top
R7  40.32,17.14 270 bottom
R8  49.53,13.34 0 bottom
SJ1  51.44,55.24 0 top
U1  57.15,3.81 180 top
U2  ACS713-20A  [SOIC8']  45.72,46.99 270 top
U3  45.09,16.51 270 bottom
U4  32.7,32.7 90 bottom
U5  18.73,32.7 90 bottom
U6  4.76,32.7 90 bottom
U$1  63.02,20.64 0 top
X1  59.69,41.75 90 top
X2  63.5,48.58 90 top
X3  21.59,11.11 0 top

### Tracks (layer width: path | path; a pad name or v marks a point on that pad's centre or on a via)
+5V  (via drill 0.61)
  Top 0.406: 53.44,69.95 L1.2 v53.34,66.99 50.48,66.99 48.9,65.41 48.9,55.24 | 48.9,55.24 SJ1.1 | v46.04,52.07 46.04,53.82 47.62,55.24 48.9,55.24
  Bottom 0.254: 4.43,29.54 4.45,29.53 | C28.1 2.41,27.17 | 32.24,29.38 32.38,29.53 | 32.38,30.5 U4.3 | C24.1 16.38,27.17 | 30.35,27.17 C20.1 | D4.2 30.8,29.53 | D5.2 16.83,29.37
  Bottom 0.406: U6.3 4.43,29.54 | 4.45,29.53 4.3,29.38 D6.2 | D6.2 2.7,28.57 2.54,28.26 C28.1 | U5.3 18.41,29.53 18.27,29.38 D5.2 16.67,28.42 16.51,28.26 C24.1 | 32.24,29.38 D4.2 30.64,28.42 30.48,28.26 C20.1 | 32.38,29.53 32.38,30.5 | C19.A 30.35,27.17 | C27.A 2.41,27.17 | C23.A 16.38,27.17 | 30.8,29.53 30.16,29.53 28.89,30.48 28.89,43.5 | 16.83,29.37 15.56,29.37 15.24,29.84 15.24,43.81 | 28.89,43.5 24.45,48.26 21.59,48.26 17.14,43.81 15.24,43.81 | D6.2 1.74,29.38 1.27,29.84 1.27,41.91 7.62,48.26 10.79,48.26 13.97,44.77 14.92,43.81 15.24,43.81 | IC2.4 57.04,63.61 53.66,66.99 v53.34,66.99 C11.A | 28.89,43.5 30.8,43.5 39.37,52.07 v46.04,52.07
  Bottom 0.61: C11.A
CAN_RX  (via drill 0.61)
  Top 0.254: 58.26,20 56.2,21.91 54.61,21.91 53.98,22.54 53.98,24.45 54.7,25.18 IC1.7 | 60.01,5.86 U1.4
  Top 0.305: 58.26,20 v58.42,19.84 | 60.01,5.86 60.01,7.62 v59.69,7.94
  Bottom 0.305: v58.42,19.84 58.42,9.21 v59.69,7.94
CAN_TX  (via drill 0.61)
  Top 0.254: 57.15,20 55.72,21.27 54.29,21.27 53.34,22.23 53.34,24.77 53.91,25.33 IC1.6
  Top 0.305: U1.1 58.42,1.91 57.15,3.17 v57.15,7.94 | v57.15,18.26 57.15,20
  Bottom 0.305: v57.15,7.94 v57.15,18.26
CHANNEL_A
  Bottom 0.254: U3.12 44.42,12.72 44.45,12.7 43.81,12.06 43.18,12.06 42.55,11.43 J3.2
CHANNEL_B
  Bottom 0.254: U3.11 J3.3
GND  (via drill 0.61, 0.89, 1.1, 1.1 pad 0.81)
  Top 0.254: v6.35,27.3 v8.89,27.3 | v20.32,27.3 v22.86,27.3 | R6.2 18,55.46 v17.78,55.24 | U1.2 60.64,3.17 | 61.28,2.54 C6.2 | IC1.5 53.1,27.7 v53.66,28.26 | IC1.20 53.1,36.28 v53.34,36.51 | v55.56,36.51 55.56,35.15 IC1.17 | v42.23,27.94 v42.23,31.11 | U2.5 43.81,45.56 44.29,46.04 49.05,46.04 49.53,46.03 C10.2 49.53,46.03 | C12.2 v47.15,39.21
  Top 0.305: 60.64,3.17 61.28,2.54 | v62.39,42.86 62.39,43.34 62.19,43.54 X1.6
  Top 0.406: C9.- 60.52,67.18 56.52,64.14 v53.34,64.14
  Top 0.813: J2.1 69.09,20.19 v69.06,20.16 | J1.1 69.09,9.4 v69.06,9.05 64.77,9.05 64.77,9.37 C7.2 64.42,10.93 C8.C 65.23,13.83 D7.A
  Top 1.778: Q4.3 32.03,45.44 v30.48,46.99 | Q6.3 18.06,45.44 v16.51,46.99 | C22.- 19.88,70.04 v17.78,67.94 | C18.- 33.84,70.04 v31.75,67.63 | Q8.3 5.36,48.93 v5.4,48.9 | v7.3,67.94 9.21,69.85 9.97,69.85 C26.-
  Bottom 0.254: C23.C 18.41,25.53 C24.2 v20.32,27.3 | C19.C 32.38,25.53 C20.2 35.72,27.3 36.35,27.94 v42.23,27.94 | v8.89,27.3 8.89,31.75 7.94,32.7 U6.9 | v22.86,27.3 22.86,31.43 21.91,32.7 U5.9 | v17.78,55.24 16.51,55.24 | C17.2 40.01,6.03 J3.1 40.01,14.61 40.64,15.24 42.23,15.24 44.45,17.46 | 44.45,17.46 44.45,19.41 U3.3 | C13.2 44.77,17.46 44.45,17.46 | v53.66,28.26 53.98,28.57 C1.2 50.16,29.85 49.21,30.8 49.21,34.92 49.53,35.24 49.53,36.99 50.01,37.47 51.12,37.47 52.07,36.51 v53.34,36.51 v55.56,36.51 | v42.23,31.11 42.23,32.7 | 42.23,32.7 U4.9 | v47.15,39.21 42.23,34.29 42.23,32.7
  Bottom 0.305: v62.39,42.86 62.39,41.75 C2.2
  Bottom 0.406: v53.34,64.14 51.44,64.14 49.85,62.55 C11.C | 53.49,64.28 v53.34,64.14 | C14.2 22.54,12.71 X3.P6 | IC2.3 56.83,61.91 56.2,62.55 55.71,62.55 D3.2 55.56,63.5 54.93,64.14 v53.34,64.14
  Bottom 0.813: v69.06,20.16 v69.06,9.05
  Bottom 1.778: v17.78,67.94 16.51,66.67 16.51,55.24 v16.51,46.99 | v31.75,67.63 30.48,66.04 v30.48,46.99 | v5.4,48.9 7.3,51.12 v7.3,67.94
  other vias: 2.54,11.43 63.66,72.07 56.67,45.88
  pour Bottom (isolate 0.406): 75,75 75,0 0,0 0,75
  pour Top (isolate 0.406, rank 2): 0,0 0,75 75,75 75,0
HALL_1  (via drill 0.61)
  Top 0.254: X3.P1 27.89,8.52 32.97,8.52 38.1,13.97 42.23,13.97 42.86,13.34 48.42,13.34 49.37,14.29 49.37,17.78 49.85,18.26 v50.64,18.26 | v61.59,26.35 61.59,30.96 59.85,32.7 57.09,32.7 IC1.15
  Bottom 0.254: v50.64,18.26 50.64,19.21 52.39,21.27 58.9,21.27 61.59,23.97 v61.59,26.35
HALL_2  (via drill 0.61)
  Top 0.254: v49.37,19.53 48.26,18.41 48.26,14.61 47.62,13.97 43.5,13.97 42.55,14.76 37.62,14.76 33.02,10.16 24.77,10.16 23.69,9.09 X3.P2 | v60.33,27.3 60.33,29.21 58.42,31.11 57.08,31.11 IC1.13
  Bottom 0.254: v49.37,19.53 51.75,21.91 58.42,21.91 60.33,23.81 v60.33,27.3
HALL_3
  Top 0.254: X3.P5 29.42,13.86 33.18,17.46 40.96,17.46 42.55,19.05 42.55,25.4 43.18,26.04 43.18,32.86 47.94,37.47 50.96,37.47 51.51,36.92 IC1.22
HSSOURCE_1  (via drill 0.61)
  Top 0.254: 33.7,40.01 Q4.4 | Q4.4 34.92,37.51 v34.92,34.29 34.92,32.49 L2.1 | 40.38,42.96 Q4.4
  Top 1.778: Q3.3 40.38,42.96
  Bottom 0.254: U4.8 34.33,34.89 v34.92,34.29 | C21.2 v30.8,40 v30.8,40.01
  pour Top (isolate 0.406, no thermals): 29.21,46.35 29.21,20.32 42.55,20.32 42.55,46.35
HSSOURCE_2  (via drill 0.61)
  Top 0.254: v16.83,40.01 19.73,40.01 Q6.4 | 26.41,42.96 Q6.4 | Q6.4 21.59,35.24 20.95,34.61 v20.95,34.29 20.95,32.17 L3.1
  Top 1.778: Q5.3 26.41,42.96
  Bottom 0.254: C25.2 v16.83,40 v16.83,40.01 | U5.8 20.36,34.89 v20.95,34.29
  pour Top (isolate 0.406, no thermals): 15.24,20.32 15.24,46.35 28.26,46.35 28.26,20.32
HSSOURCE_3  (via drill 0.61)
  Top 0.254: 6.35,30.16 6.35,30.9 L4.1 6.99,32.8 v6.99,34.29 7.62,34.97 Q8.4 | v2.86,40.01 5.75,40.01 Q8.4 | 12.44,42.96 Q8.4
  Top 1.778: Q7.3 12.44,42.96
  Bottom 0.254: U6.8 6.31,34.89 v6.99,34.29 | C29.2 v2.86,40 v2.86,40.01
  pour Top (isolate 0.406, no thermals): 1.27,20.32 1.27,46.35 14.29,46.35 14.29,20.32
INDEX/
  Bottom 0.254: U3.10 45.74,12.72 45.72,12.7 46.35,12.06 46.99,12.06 47.62,11.43 J3.4
LED_RED  (via drill 0.61)
  Top 0.254: IC1.23 50.7,36.29 v50.48,36.51 | v59.85,34.61 60.96,34.61 62.23,33.34 R2.2
  Bottom 0.254: v50.48,36.51 50.48,34.13 50.01,33.66 50.01,32.38 50.48,31.91 51.59,31.91 53.82,34.29 59.53,34.29 v59.85,34.61
LED_YELLOW
  Top 0.254: R3.2 63.18,30.8 60.38,33.6 IC1.16
LFLAG/  (via drill 0.61)
  Top 0.254: IC1.32 48.41,27.46 48.26,27.3 46.04,27.3 44.45,25.72 44.45,17.62 v46.83,15.08
  Bottom 0.254: R8.2 48.43,13.59 U3.8 46.99,13.64 46.99,14.76 v46.83,15.08
MISO  (via drill 0.61)
  Top 0.254: v48.58,26.35 49.75,26.35 IC1.1 | v55.24,22.86 55.56,22.54 57.47,22.54 58.1,23.34 61.28,23.34 66.52,28.42 69.37,28.42 70.17,29.21 70.17,34.45 67.47,36.83
  Top 0.305: 67.47,36.83 67.47,38.42 66.36,39.53 v64.29,39.53 | v63.82,37.31 63.18,36.67 59.05,36.67 58.42,37.31 X1.1
  Bottom 0.254: U3.6 46.38,20.34 46.99,20.95 47.94,20.95 48.58,21.59 48.58,24.13 | 48.58,24.13 v48.58,26.35 | v55.24,22.86 52.07,22.86 50.8,24.13 48.58,24.13
  Bottom 0.305: v64.29,39.53 64.29,37.62 v63.82,37.31
MOSI  (via drill 0.61)
  Top 0.254: v49.53,23.18 50.7,24.35 IC1.2 50.7,32.77 v50.96,33.02 | v65.25,43.5 65.25,44.77 63.5,46.51 60.48,46.51
  Top 0.305: 60.48,46.51 59.69,45.72 X1.4
  Bottom 0.254: U3.7 48.01,19.43 49.53,21.27 v49.53,23.18 | v50.96,33.02 52.7,35.08 57.78,35.08 65.25,42.23 v65.25,43.5
N$1  (via drill 0.61)
  Top 0.406: L1.1 v53.34,61.91
  Bottom 0.406: v53.34,61.91 54.61,61.91 54.78,61.77 54.93,61.62 54.93,60.64 55.08,60.49 D3.1 56.66,60.49 56.83,60.33 58.07,60.33 IC2.2
N$2
  Top 0.254: R2.1 D1.C
N$3
  Top 0.254: R3.1 D2.C
N$4
  Top 0.813: J2.4 67.92,23.94 67.31,23.34 67.31,20.64 | 67.31,20.64 67.31,13.81 67.94,13.18 68.26,13.15 J1.4 | U$1.2 67.31,20.64
N$5  (via drill 0.61)
  Top 0.305: v52.55,5.08 53.18,4.45 U1.6 | J1.2 72.7,10.65 v72.71,10.64 | v72.71,21.43 J2.2
  Top 0.406: J1.2 67.63,10.65 v66.36,10.64
  Bottom 0.305: v52.55,5.08 60.8,5.08 64.77,9.05 R4.2 66.14,10.42 v66.36,10.64 | v72.71,10.64 v72.71,21.43
N$6  (via drill 0.61)
  Top 0.305: U1.7 v52.55,3.17 | J2.3 v68.75,22.69 v68.74,22.7
  Top 0.406: J1.3 67.47,11.91 v67.32,12.05 v67.31,12.05 v67.31,12.06
  Bottom 0.305: v52.55,3.17 60.8,3.17 67.63,10 67.63,11.59 67.31,11.91 v67.31,12.06 | R4.1 67.25,12.12 v67.31,12.06 | v68.74,22.7 67.31,21.27 v67.31,12.06
N$7  (via drill 0.61)
  Top 0.254: IC1.11 55.81,29.6 v55.56,29.84
  Bottom 0.254: 59.37,29.84 v55.56,29.84
  Bottom 0.406: C5.1 62.55,34.92 62.08,34.46 Q1.3 60.64,32.28 60.01,31.65 60.01,30.48 59.37,29.84
N$8
  Bottom 0.254: U5.6 18.4,36.2 | 18.4,36.2 C25.1 | D5.1 16.67,35.72 17.14,36.2 18.4,36.2
N$9  (via drill 0.61)
  Top 0.254: IC1.10 55.78,28.8 v55.56,28.57
  Bottom 0.254: 56.52,28.57 v55.56,28.57
  Bottom 0.406: C4.1 65.82,30.58 Q1.1 64.28,29.68 63.5,28.89 59.37,28.89 59.05,28.57 v55.56,28.57
N$10
  Bottom 0.254: U4.6 32.37,36.2 | 32.37,36.2 C21.1 | D4.1 30.64,35.72 31.11,36.2 32.37,36.2
N$11
  Bottom 0.254: R7.2 41.7,16.3 43.81,18.41 43.81,19.41 U3.2
  Bottom 0.406: R7.2 39.47,16.3 39.05,15.88 39.05,15.24 38.68,14.87 Q2.3 37.3,13.48 C16.1
N$12  (via drill 0.61)
  Top 0.254: v37.78,46.99 37.78,45.5 Q4.1
  Bottom 0.254: U4.4 31.63,30.52 31.59,30.48 30.16,30.48 29.84,30.8 29.84,41.43 35.56,46.99 v37.78,46.99
N$13  (via drill 0.61)
  Top 0.254: v35.88,45.72 35.88,48.48 Q3.1
  Bottom 0.254: U4.7 33.03,36.21 33.66,36.83 33.66,43.5 v35.88,45.72
N$14
  Bottom 0.254: R7.1 41.17,18 42.61,19.43 U3.1
  Bottom 0.406: R7.1 35.08,18 | 35.08,18 33.39,18 33.18,17.78 33.18,17.3 C15.1 | Q2.1 35.09,17.69 35.08,18
N$15
  Top 1.778: F1.2 X2.P1
N$16
  Top 0.254: U2.6 45.09,43.34 47.15,41.12 48.1,41.12 C12.1
N$17  (via drill 0.61)
  Top 0.254: v23.81,46.99 23.81,45.5 Q6.1
  Bottom 0.254: U5.4 16.23,30.52 15.88,30.8 15.88,41.27 21.59,46.99 v23.81,46.99
N$18  (via drill 0.61)
  Top 0.254: v21.91,45.72 21.91,48.48 Q5.1
  Bottom 0.254: U5.7 19.06,36.21 19.68,36.83 19.68,43.18 v21.91,45.72
N$19  (via drill 3.2 pad 5.08)
  other vias: 3,3
N$20
  Bottom 0.254: U6.6 4.43,36.2 | 4.43,36.2 4.43,38.09 C29.1 | D6.1 2.7,35.72 3.17,36.2 4.43,36.2
N$21  (via drill 0.61)
  Top 0.254: v9.84,46.99 9.84,45.5 Q8.1
  Bottom 0.254: U6.4 2.18,30.52 1.91,30.8 1.91,41.27 7.62,46.99 v9.84,46.99
N$22  (via drill 0.61)
  Top 0.254: v7.94,45.72 7.94,48.48 Q7.1
  Bottom 0.254: U6.7 5.09,36.21 5.71,36.83 5.71,43.5 v7.94,45.72
N$23  (via drill 3.2 pad 5.08)
  other vias: 72,3
N$24  (via drill 3.2 pad 5.08)
  other vias: 72,72
N$25  (via drill 3.2 pad 5.08)
  other vias: 3,72
N$26  (via drill 3.2 pad 5.08)
  other vias: 3,55
N$27  (via drill 3.2 pad 5.08)
  other vias: 43,40
PWM_H_1  (via drill 0.61)
  Top 0.254: IC1.29 44.85,30.4 v44.77,30.48
  Bottom 0.254: v44.77,30.48 43.81,30.48 43.18,29.84 35.24,29.84 34.61,30.48 33.71,30.48 U4.1
PWM_H_2  (via drill 0.61)
  Top 0.254: v44.77,27.94 44.77,28.89 45.4,29.53 48.34,29.53 IC1.30
  Bottom 0.254: U5.1 20.02,30.47 21.91,28.57 21.91,24.77 24.45,22.7 33.81,22.7 38.1,26.83 43.02,26.83 44.13,27.94 v44.77,27.94
PWM_H_3  (via drill 0.61)
  Top 0.254: IC1.8 55.51,26.41 55.56,26.35 v56.83,26.35
  Bottom 0.254: U6.1 5.71,30.48 6.04,30.49 6.35,30.16 7.94,28.57 7.94,24.77 11.59,21.43 34.61,21.43 38.42,25.08 44.61,25.08 47.78,27.94 50.48,27.94 51.91,26.35 v56.83,26.35
PWM_L_1  (via drill 0.61)
  Top 0.254: v45.4,31.75 46.04,31.11 48.33,31.11 IC1.28
  Bottom 0.254: U4.2 33.03,29.52 33.34,29.21 45.09,29.21 45.72,29.84 45.72,31.43 v45.4,31.75
PWM_L_2  (via drill 0.61)
  Top 0.254: IC1.27 47.06,32 v46.35,32.7
  Bottom 0.254: U5.2 19.06,29.2 19.37,28.89 20.64,28.89 21.27,28.26 21.27,24.45 23.81,22.07 34.13,22.07 38.1,25.88 44.29,25.88 45.72,27.3 45.72,29.05 46.35,29.69 v46.35,32.7
PWM_L_3  (via drill 0.61)
  Top 0.254: v46.35,25.08 v49.53,25.08 | v56.52,23.81 56.83,23.81 57.78,24.77 57.78,27.62 57.41,28 IC1.9
  Bottom 0.254: U6.2 5.09,29.52 5.08,29.5 5.4,29.21 5.71,28.89 6.67,28.89 7.3,28.26 7.3,24.45 10.95,20.8 34.92,20.8 36.67,22.38 45.24,22.38 46.35,23.5 v46.35,25.08 | v49.53,25.08 51.12,25.08 52.39,23.81 v56.52,23.81
RESET  (via drill 0.61)
  Top 0.254: C3.1 54.13,41.75 53.98,41.59 R1.1 54.19,40.32 52.39,40.32 52.23,40.48 v52.23,43.18 | IC1.31 47.05,28.8 v46.74,28.48
  Top 0.305: 54.19,40.32 55.72,40.32 56.83,41.43 60.64,41.43 60.96,41.12 X1.5
  Bottom 0.254: v52.23,43.18 52.23,42.39 51.91,42.07 47.31,37.15 47.31,29.05 v46.74,28.48
SCK  (via drill 0.61)
  Top 0.254: IC1.12 57.87,30.4 59.05,29.21 v59.05,24.92 61.59,24.92 65.88,29.21 68.9,29.21 69.37,29.69 69.37,33.97 66.67,36.51
  Top 0.305: 66.67,36.51 66.67,38.1 66.36,38.42 63.5,38.42 62.87,37.78 60.17,37.78 59.69,38.26 X1.3
  Bottom 0.254: U3.5 45.74,20.61 45.72,20.64 46.67,21.59 47.62,21.59 47.94,21.91 47.94,24.13 47.47,24.45 47.47,26.67 48.1,27.3 50.16,27.3 52.39,24.92 v59.05,24.92
SHUNT_FILT  (via drill 0.61)
  Top 0.254: IC1.18 54.7,36.1 54.61,36.2 54.61,37.31 v54.45,37.47 | v51.28,38.42 50.48,39.21 50.48,41.91 50.01,42.39 47.15,42.39 46.35,43.18 U2.7
  Bottom 0.254: v54.45,37.47 52.23,37.47 v51.28,38.42
SS/  (via drill 0.61)
  Top 0.254: v46.99,22.54 47.94,22.54 48.26,22.23 50.16,22.23 51.44,23.5 51.44,26.43 IC1.3
  Bottom 0.254: U3.4 45.09,20.95 46.67,22.54 v46.99,22.54
STANDBY  (via drill 0.61)
  Top 0.254: v48.58,36.35 48.58,33.76 IC1.25 47.37,33.6 46.99,33.97 45.72,33.97 43.81,32.07 43.81,24.45 43.5,24.13 v43.5,23.5 | 52.39,20.32 51.44,21.27 46.35,21.27 45.4,22.23 v45.4,23.97
  Top 0.305: U1.8 52.39,1.91 51.12,3.02 51.12,7.46 52.39,8.89 52.39,20.32
  Top 0.406: v60.33,55.88 58.1,55.88 55.88,53.66 55.88,50.64 55.56,50.16 55.56,46.67 54.93,46.04 v54.93,45.72
  Bottom 0.254: 54.93,43.81 48.58,37.15 v48.58,36.35 | v45.4,23.97 44.93,23.97 44.45,23.5 v43.5,23.5
  Bottom 0.406: IC2.5 59.78,65.32 60.33,64.77 v60.33,55.88 | 54.93,43.81 v54.93,45.72
TEMP  (via drill 0.61)
  Top 0.254: IC1.14 55.95,32 55.72,32.23 55.72,33.81 57.63,35.72
  Top 0.305: 57.63,35.72 61.75,35.72 61.91,35.56 64.77,35.56 65.41,36.2 v65.41,37.31
  Top 0.406: R6.1 v19.68,51.44 | v66.36,41.75 66.36,45.09 62.71,48.58 62.71,49.69 62.07,50.32 58.9,50.32 v57.15,52.23
  Bottom 0.254: v19.68,51.44 19.68,50.8 20.95,49.53 24.13,49.53 28.57,45.09 31.11,45.09 39.37,53.02 50.27,53.02 R5.1 50.32,52.49 50.32,51.59 50.8,50.96 53.82,50.96 55.09,52.23 v57.15,52.23 | v65.41,37.31 66.36,38.26 v66.36,41.75
VCC  (via drill 0.61)
  Top 0.254: U2.8 48.18,43.89 48.58,43.5 C10.1 | v41.91,12.7 49.53,12.7 50.16,12.06 J3.5 | 61.59,4.45 61.91,4.76 C6.1 | SJ1.2 52.23,52.55 v53.34,52.55 | D2.A D1.A 71.75,33.65 71.75,34.13 68.1,37.47 68.1,39.21 66.99,40.32 65.56,40.32 64.77,41.12 | v56.99,38.1 56.67,38.1 56.04,38.73 54.08,38.73 R1.2 | 52.3,39.13 52.23,39.21 | v54.45,33.18 54.29,33.18 53.74,33.73
  Top 0.305: 61.59,4.45 U1.3 | 64.77,41.12 63.66,42.23 v63.66,44.77 | v54.45,6.99 54.45,5.73 U1.5 | X1.2 v58.42,45.56
  Top 0.406: 52.3,33.66 IC1.21 52.3,38.73 | 52.3,33.66 IC1.4 52.3,25.16 52.7,24.77 52.7,21.27 v53.97,20.01 | IC1.19 53.91,33.9 53.74,33.73 53.66,33.66 52.3,33.66 | C10.1 50.8,43.5 | 50.8,43.5 50.8,42.39 51.28,41.91 51.28,40.16 52.23,39.21 | 52.3,38.73 53.98,38.73 R1.2 | 50.8,43.5 50.8,43.81 v52.23,45.24 | v47.94,51.91 51.75,51.91 52.23,52.55 52.23,55.21 SJ1.2 | 52.3,38.73 52.3,39.13 | C6.1 v64.14,4.45
  Top 0.813: U$1.1 60.81,20.32 D7.C 60.81,13.83 C8.A 61.62,10.61 C7.1 61.91,4.76
  Bottom 0.254: C17.1 48.9,6.35 50.16,7.62 | v41.91,12.7 42.8,13.59 U3.14 U3.13 43.81,13.61 43.81,15.24 44.45,16.04 48.26,16.03 48.58,15.56 C13.1 | v54.45,6.99 53.66,7.62 51.12,7.62 50.16,7.62 | 50.16,7.62 J3.5 50.16,12.06 50.38,12.28 R8.1 51.75,13.34 | v53.34,52.55 R5.2 | C2.1 60.01,39.69 58.42,38.1 v56.99,38.1 | C1.1 53.98,32.7 v54.45,33.18
  Bottom 0.305: C13.1 51.28,15.56 53.98,18.26 53.98,20.32 v53.97,20.01 | v58.42,45.56 59.85,45.56 | 59.85,45.56 62.87,45.56 v63.66,44.77 | C2.1 60.01,45.41 59.85,45.56
  Bottom 0.406: C14.1 20.64,9.51 X3.P3 19.49,3.05 22.07,0.95 40.96,0.95 41.91,1.9 C17.1 | v52.23,45.24 52.23,47.31 48.74,50.96 v47.94,51.91 | v64.14,4.45 61.75,2.06 51.59,2.06 51.28,2.38 51.28,7.46 51.12,7.62
VDD  (via drill 0.61)
  Top 0.406: C9.+ 67.12,59.18 66.67,59.05 59.37,59.05 v56.83,56.52 54.93,54.61 54.93,51.28 54.29,50.32 54.14,50.17 F1.1
  Bottom 0.61: IC2.1 58.19,57.86 v56.83,56.52
  pour Top (no thermals): 46.35,50.8 54.61,50.8 54.61,46.99 46.35,46.99
VDD_HS
  pour Top (isolate 0.406, no thermals): 1.27,47.31 1.27,66.04 45.09,66.04 45.09,47.31
WINDING_1
  Top 1.778: X3.P7 19.49,15.52 20.8,16.83 27.78,16.83 31.75,20.8 35.14,20.8 L2.2
WINDING_2
  Top 1.778: L3.2 17.2,20.85 15.29,19.1 X3.P8
WINDING_3
  Top 1.778: L4.2 7.62,12.86 12.12,8.36 X3.P4

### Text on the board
Bottom: Weklin MotorBoard v2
